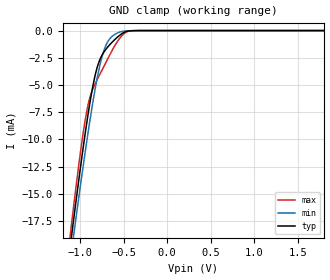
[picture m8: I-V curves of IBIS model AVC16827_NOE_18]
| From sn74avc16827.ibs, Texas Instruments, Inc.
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[Model]   AVC16827_NOE_18
Model_type  Input
Vinl=0.5775
Vinh=1.2675
| variable   typ   min   max
C_comp   2.39pF   1.59pF   2.73pF
[Temperature Range]   40   100   -40
| Ambient temperature   25   85   -40
[Voltage range]   1.8   1.65   1.95
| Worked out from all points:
|   GND clamp passes 1 mA (typ) near -0.62 V on its own axis
[GND Clamp]
| AVC16827_NOE_18
|   Voltage   I(typ)   I(min)   I(max)
-1.8V     -66.75mA   -65.67mA   -69.43mA
-1.11V    -19.59mA   -20.97mA   -18.51mA
-1.095V   -18.63mA   -20.05mA   -17.49mA
-1.07V    -17.06mA   -18.55mA   -15.82mA
-995mV    -12.48mA   -14.14mA   -11.08mA
-935mV    -9.059mA   -10.77mA   -7.878mA
-890mV    -6.731mA   -8.379mA   -6.205mA
-830mV    -4.188mA   -5.47mA    -4.924mA
-725mV    -1.948mA   -1.787mA   -3.26mA
-605mV    -848.6uA   -366.4uA   -1.429mA
-420mV    -20.38uA   -15.02uA   -24.05uA
1.8V      256.7pA    930.1pA    14.18pA
